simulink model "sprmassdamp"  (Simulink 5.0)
settings: Solver=ode45  StartTime=0.0  StopTime=25  RelTol=1e-6
libraries: simulink x1

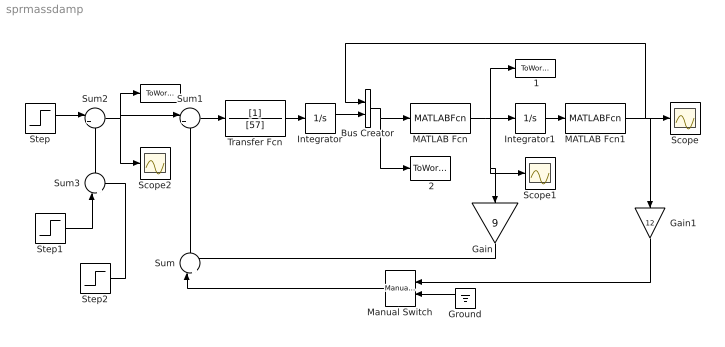
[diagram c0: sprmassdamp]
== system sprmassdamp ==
  " " : ToWorkspace  VariableName=u  SampleTime=-1  SaveFormat=Array
  " 1" : ToWorkspace  VariableName=v  SampleTime=-1  SaveFormat=Array
  " 2" : ToWorkspace  VariableName=x  SampleTime=-1  SaveFormat=Array
  Bus Creator : BusCreator  Inputs=2
  Gain : Gain  Orientation=down  Gain=9
  Gain1 : Gain  Orientation=down  Gain=12
  Ground : Ground  Orientation=left
  Integrator : Integrator
  Integrator1 : Integrator
  MATLAB Fcn : MATLABFcn  MATLABFcn=batas
  MATLAB Fcn1 : MATLABFcn  MATLABFcn=satamp
  Manual Switch : simulink/Signal Routing/Manual Switch  Orientation=left  sw=0  action=0
  Scope : Scope
  Scope1 : Scope
  Scope2 : Scope
  Step : Step  Time=0  After=100  SampleTime=0
  Step1 : Step  Time=2  After=-200  SampleTime=0
  Step2 : Step  Time=5  After=100  SampleTime=0
  Sum : Sum  Orientation=up  Inputs=|++
  Sum1 : Sum  Inputs=|+-
  Sum2 : Sum  Inputs=|++
  Sum3 : Sum  Orientation=up  Inputs=|++
  Transfer Fcn : TransferFcn  Denominator=[57]
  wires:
  Transfer Fcn/1 -> Integrator/1
  Integrator1/1 -> MATLAB Fcn1/1
  Gain/1 -> Sum/2
  Integrator/1 -> Bus Creator/2
  MATLAB Fcn/1 -> Integrator1/1, Gain/1, Scope1/1, " 1"/1
  Bus Creator/1 -> MATLAB Fcn/1, " 2"/1
  Sum1/1 -> Transfer Fcn/1
  Step/1 -> Sum2/1
  Sum2/1 -> Sum1/1, Scope2/1, " "/1
  Sum/1 -> Sum1/2
  MATLAB Fcn1/1 -> Scope/1, Gain1/1, Bus Creator/1
  Sum3/1 -> Sum2/2
  Step1/1 -> Sum3/1
  Step2/1 -> Sum3/2
  Gain1/1 -> Manual Switch/1
  Manual Switch/1 -> Sum/1
  Ground/1 -> Manual Switch/2
